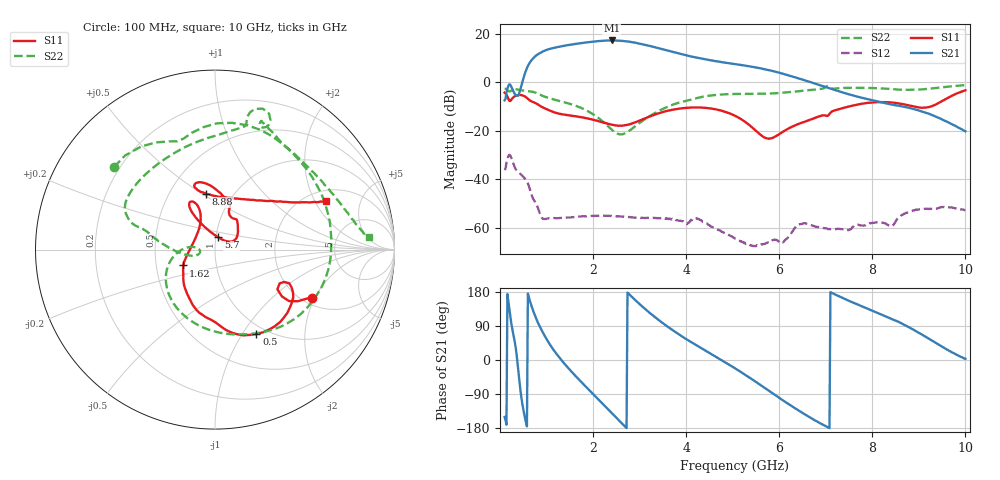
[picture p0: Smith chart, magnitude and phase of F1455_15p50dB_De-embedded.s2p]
! Integrated Device Technology
! Corporate Headquarters
! 6024 Silver Creek Valley Road
! San Jose, CA 95138  USA
! Phone:  1-408-284-8200
! Toll Free:  1-800-223-1366
! Webpage:  http://www.idt.com/
! Timing and RF Division
! 515 Groton Road, Suite 102
! Westford, MA 01886-6024
! Device:  F1455
! Description: 6-bit 0.5 dB Transmit Variable Gain Amplifier
! Frequency:  1400.0 -  2300.00 MHz
! Package:  6x6 mm Thin QFN Plastic Package: 28 pin
! State:  31
! Atten State:  15.5 dB
! Voltage:  +5.00 Volts
! Current:  217.625 mA
! Data:  The device was measured on a the F1455 evaluation board which has
!  individual transmission lines to the RF pins.  Data was collected
!  using a calibrated network analyzer.  The evaluation board was
!  de-embedded using a TRL calibration technique.
!  The reference plane is the edge of the package pin.
!  Pin  1 = CSb
!  Pin  2 = DATA
!  Pin  3 = CLK
!  Pin  4 = RSET
!  Pin  5 = GND
!  Pin  6 = RFIN  = Port 1
!  Pin  7 = GND
!  Pin  8 = NC
!  Pin  9 = NC
!  Pin 10 = NC
!  Pin 11 = NC
!  Pin 12 = NC
!  Pin 13 = NC
!  Pin 14 = /STBY
!  Pin 15 = GND
!  Pin 16 = RFOUT  = Port 2
!  Pin 17 = GND
!  Pin 18 = NC
!  Pin 19 = NC
!  Pin 20 = NC
!  Pin 21 = GND
!  Pin 22 = NC
!  Pin 23 = GND
!  Pin 24 = NC
!  Pin 25 = NC
!  Pin 26 = NC
!  Pin 27 = GND
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# GHz S dB R 50
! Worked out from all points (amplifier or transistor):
!   496 points, 100 MHz to 10 GHz, reference 50 ohm
!   highest |S21| = 17.1 dB at 2.4 GHz (marker M1)
!   |S21| within 3 dB of that: 1.173 GHz to 3.373 GHz (2.2 GHz wide, 96.8 % of centre)
!   unconditionally stable (mu >= 1): start of sweep to end of sweep
!   at 1.74 GHz: K = 41.01, MAG = 16.6 dB, |S12| = -55.4 dB
!   at 5.06 GHz: K = 236.87, MAG = 9.2 dB, |S12| = -64.6 dB
!   at 10 GHz: K = 315.61, MAG = -11.8 dB, |S12| = -52.8 dB
!   S11 on the Smith chart (normalised r, x): 100 MHz: 2.25, -1.91; 500 MHz: 0.89, -1.16; 1.62 GHz: 0.69, -0.13; 5.7 GHz: 1.03, +0.14; 8.88 GHz: 0.75, +0.52; 10 GHz: 2.47, +2.47
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0.1  -4.37 -26.4  -7.51 -150.3  -36.28 46.1  -2.77 140.7
0.26  -6.85 -24.4  -2.63 85.3  -32.10 -76.3  -3.29 95.5
0.38  -5.43 -41.2  -5.66 -10.3  -36.85 -115.2  -3.12 57.5
0.5  -5.62 -63.8  1.29 -129.5  -39.02 -153.4  -3.49 27.4
0.68  -7.98 -91.3  9.04 141.7  -46.50 142.5  -3.92 -14.2
0.82  -9.31 -109.3  11.50 97.5  -52.09 119.0  -4.80 -45.7
0.96  -10.82 -123.1  12.93 64.1  -56.47 124.6  -6.03 -70.9
1.28  -13.09 -142.6  14.58 6.0  -56.10 94.7  -7.81 -114.4
1.62  -14.10 -153.5  15.70 -41.7  -55.64 65.2  -9.73 -147.0
1.76  -14.53 -157.4  16.08 -59.7  -55.35 55.0  -10.79 -157.9
2.08  -15.90 -168.2  16.82 -99.6  -55.16 35.4  -14.31 -178.6
2.4  -17.57 171.7  17.14 -139.8  -55.16 18.7  -19.59 173.9
2.78  -17.47 136.2  16.61 173.1  -55.62 3.1  -20.07 -163.4
3.08  -15.26 118.0  15.51 138.8  -56.01 -6.4  -15.74 -169.7
3.4  -12.96 111.6  14.00 106.4  -56.06 -17.2  -12.05 178.2
4.08  -10.54 115.6  10.65 49.3  -57.49 -31.4  -7.38 163.6
5.06  -14.00 120.6  7.36 -22.7  -64.61 -75.5  -4.91 148.5
5.7  -22.98 75.4  5.24 -74.6  -66.60 -51.9  -4.81 122.3
6.7  -15.29 42.1  -0.21 -154.5  -59.02 -133.6  -3.22 78.5
8.36  -8.36 107.1  -9.08 111.3  -59.24 138.2  -2.84 62.5
8.88  -10.05 98.9  -11.08 80.1  -52.88 133.7  -3.19 42.1
10  -3.42 23.8  -20.31 3.3  -52.79 54.3  -1.29 4.6
